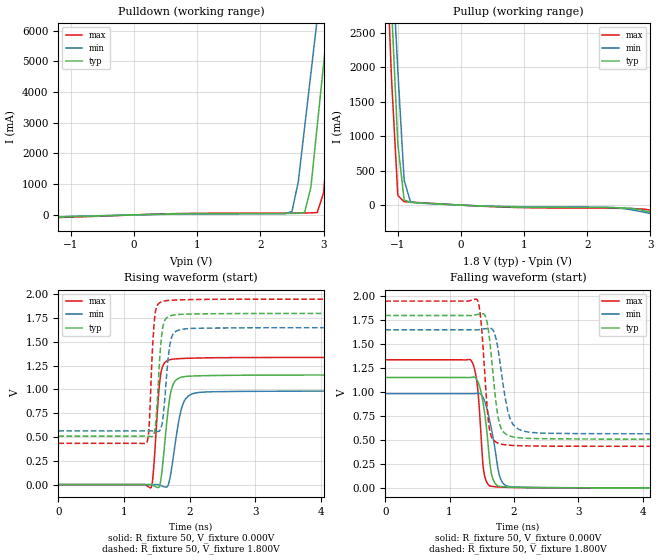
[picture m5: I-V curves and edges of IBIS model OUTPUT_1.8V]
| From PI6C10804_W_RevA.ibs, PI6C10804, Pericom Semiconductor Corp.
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[Model]   OUTPUT_1.8V
Model_type Output
Vref=1.800V
Vmeas=900mV
| variable   typ   min   max
C_comp   1.150pF   1.149pF   1.151pF
[Voltage Range]   1.8000V   1.6500V   1.9500V
[POWER Clamp Reference]   1.8000V   1.6500V   1.9500V
[GND Clamp Reference]   0.0000V   0.0000V   0.0000V
[Pullup Reference]   1.8000V   1.6500V   1.9500V
[Pulldown Reference]   0.0000V   0.0000V   0.0000V
[Temperature Range]   25   85   -40
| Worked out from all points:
|   slope of the pulldown table from 0 to 0.27 V, typ, clamps not added: 17.9 ohm
|   slope of the pullup table from 0 to 0.27 V, typ, clamps not added: 24.1 ohm
|   falling waveform, R_fixture 50, V_fixture 0.000V: 20-80 % time 120ps typ, 158ps min, 84.6ps max; typ from 1.15 V to 0 V
|   rising waveform, R_fixture 50, V_fixture 0.000V: 20-80 % time 107ps typ, 140ps min, 80.9ps max; typ from 0 V to 1.15 V
|   falling waveform, R_fixture 50, V_fixture 1.800V: 20-80 % time 124ps typ, 157ps min, 97.3ps max; typ from 1.8 V to 0.509 V
|   rising waveform, R_fixture 50, V_fixture 1.800V: 20-80 % time 72.8ps typ, 84.6ps min, 62.3ps max; typ from 0.509 V to 1.8 V
[Pulldown]
| Voltage   I(typ)   I(min)   I(max)
-1.8V     -208mA     -175.4mA   -275.2mA
-1.1V     -63mA      -56.94mA   -77.98mA
2.5V      47.95mA    115.9mA    59.49mA
2.6V      50.91mA    1.08A      60.73mA
2.7V      84.56mA    2.848A     62.8mA
2.8V      909mA      4.616A     65.58mA
2.9V      2.907A     6.384A     76.87mA
3V        4.904A     8.152A     718.7mA
3.1V      6.902A     9.921A     3.034A
3.2V      8.9A       11.69A     5.359A
3.3V      10.9A      13.46A     7.684A
3.6V      16.89A     18.76A     14.66A
[Pullup]
| Voltage   I(typ)   I(min)   I(max)
-1.8V     16.87A     16.1A      18.11A
-1.2V     4.884A     5.49A      4.162A
-1.1V     2.886A     3.721A     1.837A
-1V       887.7mA    1.952A     140.1mA
-900mV    74.54mA    358.5mA    49.47mA
-800mV    39.45mA    50.6mA     43.51mA
-700mV    33.87mA    31.3mA     38.19mA
800mV     -26.5mA    -21.99mA   -32.24mA
2.4V      -37.51mA   -33.69mA   -46.04mA
2.9V      -81.29mA   -103.1mA   -57.85mA
3.1V      -126mA     -139.4mA   -101.7mA
3.6V      -245mA     -232.9mA   -270.2mA
[Falling Waveform]
R_fixture = 50
V_fixture = 0.000V
V_fixture_min = 0.000V
V_fixture_max = 0.000V
|   Time   V(typ)   V(min)   V(max)
0s        1.152V     983.7mV    1.337V
1.34ns    1.154V     983.1mV    1.326V
1.428ns   1.126V     987.9mV    1.086V
1.492ns   990.6mV    972.7mV    506.9mV
1.54ns    803mV      912.7mV    139.6mV
1.636ns   203.9mV    659.7mV    17.97mV
1.692ns   64.52mV    462.8mV    12.49mV
1.772ns   16.54mV    134.7mV    8.495mV
1.92ns    7.894mV    14.41mV    4.893mV
9.8ns     0V         1.094uV    0V
[Rising Waveform]
R_fixture = 50
V_fixture = 0.000V
V_fixture_min = 0.000V
V_fixture_max = 0.000V
|   Time   V(typ)   V(min)   V(max)
0s        0V         0V         0V
1.415ns   -473.8uV   69.81uV    -30.02mV
1.445ns   -8.64mV    351.4uV    113.1mV
1.525ns   -30.21mV   -1.71mV    929.8mV
1.56ns    44.62mV    -9.826mV   1.162V
1.665ns   740mV      -15.22mV   1.305V
1.72ns    992.7mV    145.1mV    1.316V
1.89ns    1.131V     830.2mV    1.326V
2.1ns     1.143V     964.8mV    1.331V
10ns      1.152V     983.7mV    1.337V
[Falling Waveform]
R_fixture = 50
V_fixture = 1.800V
V_fixture_min = 1.650V
V_fixture_max = 1.950V
|   Time   V(typ)   V(min)   V(max)
0s        1.8V       1.65V      1.95V
1.43ns    1.81V      1.65V      1.964V
1.49ns    1.817V     1.656V     1.726V
1.56ns    1.785V     1.662V     1.057V
1.62ns    1.558V     1.666V     613.4mV
1.73ns    843.5mV    1.531V     474.4mV
1.8ns     622.2mV    1.229V     457.1mV
1.95ns    538.2mV    707.4mV    444.1mV
2.22ns    517mV      583.2mV    438.2mV
9.8ns     508.9mV    564.1mV    434.1mV
[Rising Waveform]
R_fixture = 50
V_fixture = 1.800V
V_fixture_min = 1.650V
V_fixture_max = 1.950V
|   Time   V(typ)   V(min)   V(max)
0s        508.9mV    564.1mV    434.1mV
1.34ns    509.1mV    564.2mV    433.4mV
1.385ns   507.2mV    564.4mV    638.2mV
1.43ns    505.3mV    564.3mV    1.374V
1.47ns    576mV      562.6mV    1.772V
1.555ns   1.431V     579.5mV    1.916V
1.6ns     1.683V     739.1mV    1.928V
1.71ns    1.775V     1.51V      1.938V
1.86ns    1.79V      1.629V     1.943V
8ns       1.8V       1.65V      1.95V
[Ramp]
| variable   typ   min   max
dV/dt_r   0.69018V/107.80p   0.58936V/140.01p   0.80172V/81.158p
dV/dt_f   0.77442V/123.51p   0.65070V/157.45p   0.90924V/97.462p
R_load = 50
